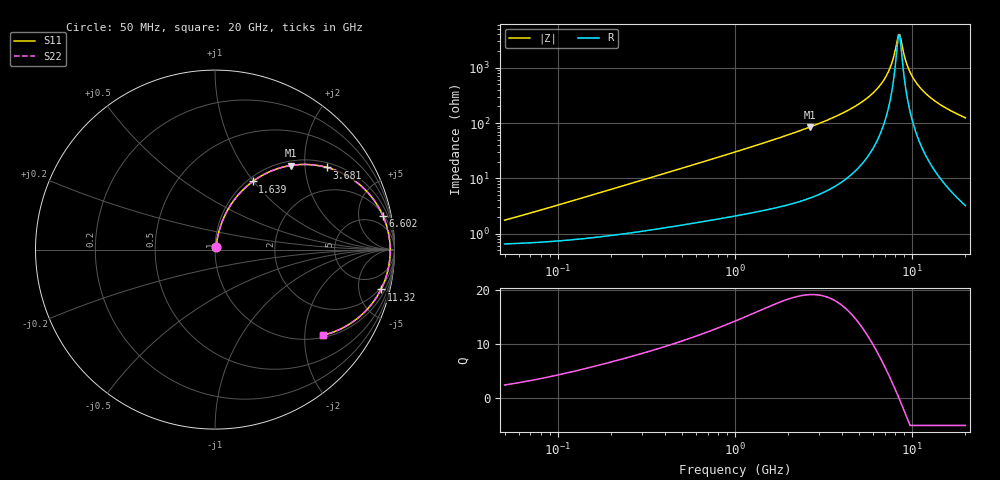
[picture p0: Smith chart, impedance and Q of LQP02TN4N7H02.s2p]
!Murata Part Number: LQP02TN4N7H02
!These Parameters are Measured in Series Mode Connection
!  o--[Z]--o
!Port1  Port2
!  o-------o
!Freq. Start=50[MHz] Stop=20[GHz], 401[Steps]
# Hz S RI R 50
!Freq.(Hz) S11(Real) S11(Imag) S21(Real) S21(Imag) S12(Real) S12(Imag) S22(Real) S22(Imag)
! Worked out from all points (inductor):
!   401 points, 50 MHz to 20 GHz, reference 50 ohm
!   read as one part in series: L = 5.13 nH near 62.6 MHz
!   highest Q = 19.2 at 2.647 GHz (marker M1), where L = 5.07 nH
!   self-resonance near 8.389 GHz
!   S11 on the Smith chart (normalised r, x): 50 MHz: 1.01, +0.03; 1.639 GHz: 1.06, +0.99; 3.681 GHz: 1.14, +2.60; 6.602 GHz: 2.26, +9.55; 11.32 GHz: 1.74, -8.07; 20 GHz: 1.06, -2.48
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5e7  0.00674 0.016  0.9933 -0.016  0.9933 -0.016  0.00674 0.016
1.364002e8  0.00982 0.0425  0.9902 -0.0425  0.9902 -0.0425  0.00982 0.0425
3.721004e8  0.0244 0.1095  0.9756 -0.1095  0.9756 -0.1095  0.0244 0.1095
1e9  0.0973 0.2635  0.9027 -0.2635  0.9027 -0.2635  0.0973 0.2635
1.639343e9  0.2099 0.3794  0.7901 -0.3794  0.7901 -0.3794  0.2099 0.3794
2.647493e9  0.4208 0.4684  0.5792 -0.4684  0.5792 -0.4684  0.4208 0.4684
2.728004e9  0.4377 0.4708  0.5623 -0.4708  0.5623 -0.4708  0.4377 0.4708
3.680849e9  0.6229 0.4578  0.3771 -0.4578  0.3771 -0.4578  0.6229 0.4578
5.194772e9  0.833 0.3371  0.167 -0.3371  0.167 -0.3371  0.833 0.3371
5.944466e9  0.8975 0.2585  0.1025 -0.2585  0.1025 -0.2585  0.8975 0.2585
6.601595e9  0.936 0.1875  0.064 -0.1875  0.064 -0.1875  0.936 0.1875
7.442007e9  0.9649 0.0987  0.0351 -0.0987  0.0351 -0.0987  0.9649 0.0987
7.784049e9  0.9712 0.064  0.0288 -0.064  0.0288 -0.064  0.9712 0.064
8.264682e9  0.9757 0.0171  0.0243 -0.0171  0.0243 -0.0171  0.9757 0.0171
8.516016e9  0.9762 -0.0065  0.0238 0.0065  0.0238 0.0065  0.9762 -0.0065
8.644534e9  0.976 -0.0183  0.024 0.0183  0.024 0.0183  0.976 -0.0183
9.178299e9  0.9724 -0.0654  0.0276 0.0654  0.0276 0.0654  0.9724 -0.0654
9.600142e9  0.9667 -0.1004  0.0333 0.1004  0.0333 0.1004  0.9667 -0.1004
1.034674e10  0.9516 -0.1573  0.0484 0.1573  0.0484 0.1573  0.9516 -0.1573
1.131968e10  0.9246 -0.2223  0.0754 0.2223  0.0754 0.2223  0.9246 -0.2223
1.438523e10  0.8128 -0.3675  0.1872 0.3675  0.1872 0.3675  0.8128 -0.3675
2e10  0.6039 -0.4764  0.3961 0.4764  0.3961 0.4764  0.6039 -0.4764
